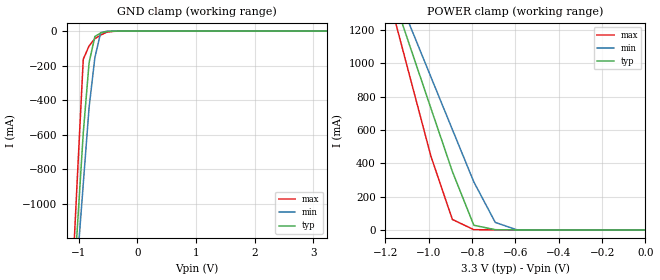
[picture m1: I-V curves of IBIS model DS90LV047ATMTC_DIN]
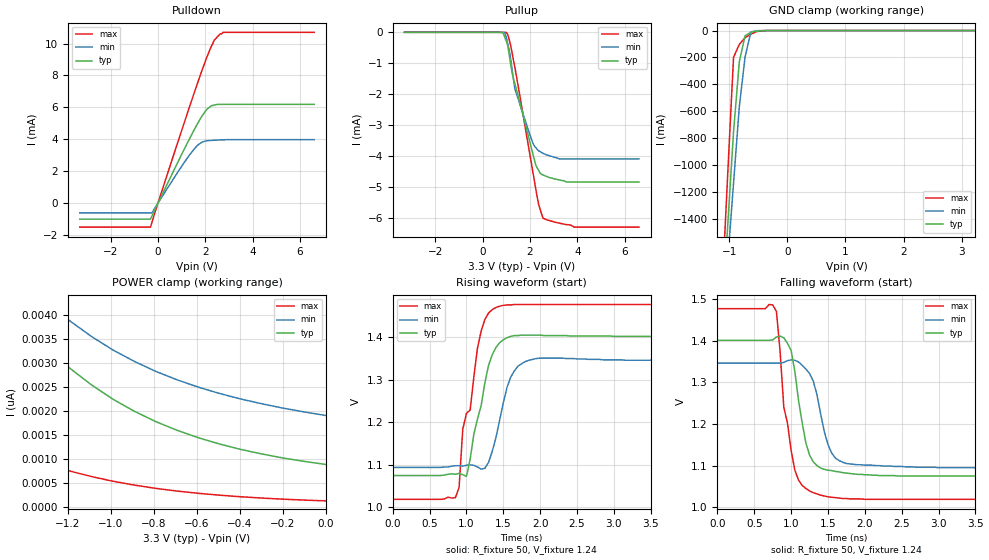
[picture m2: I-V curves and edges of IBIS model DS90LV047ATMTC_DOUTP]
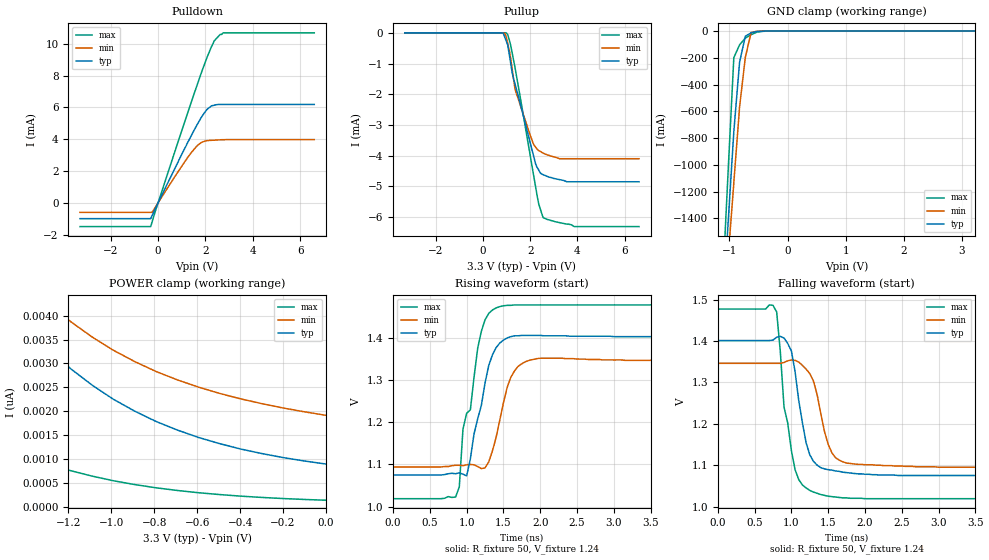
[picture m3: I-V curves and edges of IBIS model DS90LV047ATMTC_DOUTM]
|   National Semiconductor Corporation
|   Interface Products Group
|   IBIS Model of DSLVDS1047
|   16L TSSOP Package
[IBIS Ver]   3.2
[File name]   dslvds1047.ibs
[File Rev]   1.2
[Date]   7/06/04
[Source]   File originated at National Semiconductor Corporation.
   Interface Group/Analog Division. All data based on
   Empirical Measurements(Bench).
[Notes]   File created by DAK.
   Rev 1.1: In Rising Falling Tables, changes Vref
   from 3.3v to 1.2v---milt
   Rev 1.2: a new model based on a spice model simulation
   data - dglisic
[Disclaimer]
(C) Copyright National Semiconductor Corporation 1994
   All rights reserved
   National Semiconductor Corporation hereby grants
the user of this IBIS model a non-exclusive, nontransferable
license to use this IBIS model under the following terms.
Before using this IBIS model, the user should read this
license.  If the user does not accept these terms,  the
IBIS model should be returned to National within 30 days.
   The user is granted this license only to use the
IBIS model and is not granted rights to sell, load, rent,
lease or license the IBIS model in whole or in part, or in
modified form to anyone other than user. User may modify
the IBIS model to suit its specific applications but rights
to derivative works and such modifications shall belong to
National.
   This IBIS model is provided on an "AS IS" basis and
National makes absolutely no warranty with respect to the
information contained herein.NATIONAL DISCLAIMS AND CUSTOMER
WAIVES ALL WARRANTIES, EXPRESS OR IMPLIED, INCLUDING
WARRANTIES OF MERCHANTABILITY OR FITNESS FOR A PARTICULAR
PURPOSE. The entire risk as to quality and performance is
with the Customer. ACCORDINGLY, IN NO EVENT SHALL THE
COMPANY BE LIABLE FOR ANY DAMAGES, WHETHER IN CONTRACT OR
TORT,INCLUDING ANY LOST PROFITS OR OTHER INCIDENTAL,
CONSEQUENTIAL, EXEMPLARY, OR PUNITIVE DAMAGES ARISING OUT
OF THE USE OR APPLICATION OF THE IBIS model provided in
this package.Further, National reserves the right to make
changes without notice to any product herein to improve
reliability, function, or design. National does not convey
any license under patent rights or any other intellectual
property rights, including those of third parties.
   National is not obligated to provide maintenance or support
for the licensed IBIS model.
Contact National at ATTN:INTERFACE APPLICATIONS/IBIS MODELS
   5 Foden Road, M/S 03-03
   South Porltand, ME 04106
   (207) 541-6031
[Copyright]   Copyright 1994, National Semiconductor, All Rights Reserved
[Component]   DSLVDS1047
[Manufacturer]  National Semiconductor Corp
[Package]
|   typ   min   max
R_pkg   91m   78m   115m
L_pkg   2.49n   2.15n   3.12n
C_pkg   0.086p   0.076p   0.109p
[Pin]   signal_name   model_name   R_pin   L_pin   C_pin
1   EN   DS90LV047ATMTC_EN   113m   3.053n   .108p
2   DIN1   DS90LV047ATMTC_DIN   91m   2.494n   .083p
3   DIN2   DS90LV047ATMTC_DIN   80m   2.218n   .079p
4   VDD   POWER   78m   2.157n   .076p
5   GND   GND   79m   2.183n   .077p
6   DIN3   DS90LV047ATMTC_DIN   84m   2.318n   .078p
7   DIN4   DS90LV047ATMTC_DIN   93m   2.550n   .083p
8   EN*   DS90LV047ATMTC_EN   108m   2.984n   .107p
9   DOUT4-   DS90LV047ATMTC_DOUTM  115m   3.121n   .109p
10   DOUT4+   DS90LV047ATMTC_DOUTP   93m   2.551n   .083p
11   DOUT3+   DS90LV047ATMTC_DOUTP   81m   2.237n   .079p
12   DOUT3-   DS90LV047ATMTC_DOUTM   78m   2.152n   .076p
13   DOUT2-   DS90LV047ATMTC_DOUTM   79m   2.173n   .076p
14   DOUT2+   DS90LV047ATMTC_DOUTP   83m   2.291n   .078p
15   DOUT1+   DS90LV047ATMTC_DOUTP   90m   2.480n   .083p
16   DOUT1-   DS90LV047ATMTC_DOUTM  106m   2.914n   .106p
[Diff_pin]   inv_pin   vdiff   tdelay_typ   tdelay_min   tdelay_max
10   9   0.7   0   0   1.7ns
11   12   NA   0   0   0
14   13   NA   0   0   0
15   16   NA   0   0   0
| Models and submodels in the file (4): DS90LV047ATMTC_DIN (Input), DS90LV047ATMTC_EN (Input), DS90LV047ATMTC_DOUTP (3-state), DS90LV047ATMTC_DOUTM (3-state)
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[Model]   DS90LV047ATMTC_DIN
Model_type Input
Vinh=2.0
Vinl=0.8
|   TYP   MIN   MAX
C_comp   3p   3p   3p
[Temperature Range] 25   85   -40
[Voltage Range]   3.30   3.00   3.60
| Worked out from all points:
|   GND clamp passes 1 mA (typ) near -0.44 V on its own axis
|   POWER clamp passes 1 mA (typ) near -0.65 V on its own axis
[GND Clamp]
|V(groundclamp)   I(typ)   I(min)   I(max)
-3.3V     -13.98A    -11.83A    -17.63A
-1.122V   -1.669A    -1.777A    -1.526A
-1.023V   -1.129A    -1.331A    -837mA
-924mV    -590.8mA   -886.6mA   -163.5mA
-825mV    -184mA     -443.7mA   -85.99mA
-726mV    -31.28mA   -153.9mA   -44.23mA
-627mV    -11.3mA    -9.068mA   -22.94mA
-528mV    -2.886mA   -1.123mA   -6.914mA
-330mV    -102.6uA   -43.64uA   -229.3uA
3.234V    1.855uA    1.074uA    3.371uA
[POWER Clamp]
|V(table)   I(typ)   I(min)   I(max)
-3.267V   9.584A     8.291A     11.75A
-1.188V   1.491A     1.55A      1.416A
-1.089V   1.11A      1.233A     928.2mA
-990mV    729.5mA    917.3mA    441.9mA
-891mV    350.5mA    602.3mA    63.05mA
-792mV    28.24mA    288.1mA    1.817mA
-693mV    1.617mA    45.27mA    453.5uA
-594mV    118.9uA    1.221mA    66.77uA
0V        857.1pA    1.83nA     132.3pA
[Model]   DS90LV047ATMTC_DOUTP
Model_type 3-state
Enable Active-High
Polarity Non-Inverting
Vref=1.21
Vmeas=1.21
Rref=50   | 100 Ohms Across Outputs OUTP and OUTM
Cref=0p
|   TYP   MIN   MAX
C_comp   2.5p   2p   3.5p
[Temperature Range] 25   85   -40
[Voltage Range]   3.30   3.00   3.60
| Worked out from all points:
|   slope of the pulldown table from 0 to 0.495 V, typ, clamps not added: 327 ohm
|   GND clamp passes 1 mA (typ) near -0.42 V on its own axis
|   falling waveform, R_fixture 50, V_fixture 1.24: 20-80 % time 184ps typ, 203ps min, 183ps max; typ from 1.4 V to 1.07 V
|   rising waveform, R_fixture 50, V_fixture 1.24: 20-80 % time 231ps typ, 209ps min, 240ps max; typ from 1.07 V to 1.4 V
[Pullup]
|Vtable   I(typ)   I(min)   I(max)
-3.3V     1.3nA      2.13nA     2.37nA
800mV     -1.95uA    -4.2uA     2.12nA
988mV     -265uA     -130uA     1.03nA
1.05V     -391uA     -339uA     -55.9uA
1.175V    -986uA     -810uA     -399uA
1.362V    -1.67mA    -1.84mA    -1.14mA
2.112V    -3.91mA    -3.57mA    -4.49mA
2.238V    -4.29mA    -3.73mA    -5.05mA
2.362V    -4.47mA    -3.84mA    -5.57mA
2.55V     -4.62mA    -3.92mA    -6.02mA
3.862V    -4.85mA    -4.1mA     -6.31mA
6.6V      -4.85mA    -4.1mA     -6.31mA
[Pulldown]
|V(pulldown)   I(typ)   I(min)   I(max)
-3.3V     -1mA       -603uA     -1.5mA
-313mV    -1mA       -603uA     -1.5mA
-250mV    -796uA     -603uA     -1.19mA
875mV     2.67mA     2.03mA     3.98mA
1.625V    4.85mA     3.55mA     7.31mA
1.812V    5.34mA     3.78mA     8.12mA
2V        5.75mA     3.89mA     8.88mA
2.25V     6.1mA      3.93mA     9.81mA
2.375V    6.14mA     3.94mA     10.2mA
2.625V    6.19mA     3.96mA     10.6mA
2.75V     6.19mA     3.97mA     10.7mA
6.6V      6.19mA     3.98mA     10.7mA
[GND Clamp]
|V(groundclamp)   I(typ)   I(min)   I(max)
-3.3V     -17.79A    -15.11A    -22.31A
-1.122V   -2.13A     -2.273A    -1.936A
-1.023V   -1.44A     -1.703A    -1.057A
-924mV    -751.6mA   -1.134A    -198.9mA
-825mV    -232.9mA   -567.3mA   -103.3mA
-726mV    -38.72mA   -196.7mA   -52.72mA
-627mV    -13.96mA   -11.49mA   -27.64mA
-528mV    -3.584mA   -1.412mA   -8.348mA
-330mV    -123.4uA   -52.37uA   -268.9uA
3.234V    857.1pA    2.099nA    93.12pA
[POWER Clamp]
|V(table)   I(typ)   I(min)   I(max)
-3.267V   46.62nA    40.29nA    20.01nA
-2.277V   12.92nA    12.82nA    4.536nA
-2.178V   11.26nA    11.38nA    3.87nA
-1.98V    8.554nA    9.002nA    2.81nA
-1.881V   7.457nA    8.027nA    2.393nA
-1.683V   5.654nA    6.409nA    1.724nA
-1.485V   4.298nA    5.176nA    1.239nA
-1.287V   3.289nA    4.247nA    889pA
-1.089V   2.545nA    3.553nA    639.8pA
-891mV    2.001nA    3.039nA    463.6pA
-495mV    1.32nA     2.372nA    253.7pA
0V        893pA      1.913nA    134.7pA
[Ramp]
|   TYP   MIN   MAX
dV/dt_r   196mV/.233ns   153mV/.244ns   276mV/.211ns
dV/dt_f   196mv/.190ns   153mV/.216ns   276mV/.180ns
R_load=50
[Falling Waveform]
R_fixture=50
V_fixture=1.24
V_fixture_min=1.22
V_fixture_max=1.25
|Time   V(typ)   V(min)   V(max)
0s        1.401V     1.346V     1.477V
800ps     1.409V     1.346V     1.47V
850ps     1.411V     1.346V     1.373V
900ps     1.407V     1.348V     1.24V
1ns       1.376V     1.354V     1.135V
1.1ns     1.256V     1.349V     1.065V
1.25ns    1.125V     1.321V     1.039V
1.5ns     1.089V     1.15V      1.025V
1.7ns     1.083V     1.108V     1.021V
4.95ns    1.075V     1.094V     1.019V
[Rising Waveform]
R_fixture=50
V_fixture=1.24
V_fixture_min=1.22
V_fixture_max=1.25
|Time   V(typ)   V(min)   V(max)
0s        1.075V     1.094V     1.019V
850ps     1.078V     1.098V     1.023V
900ps     1.08V      1.098V     1.047V
1ns       1.073V     1.099V     1.221V
1.05ns    1.113V     1.1V       1.229V
1.15ns    1.208V     1.095V     1.375V
1.4ns     1.376V     1.164V     1.47V
1.6ns     1.402V     1.306V     1.476V
1.85ns    1.405V     1.346V     1.477V
4.95ns    1.401V     1.346V     1.477V
[Model]   DS90LV047ATMTC_DOUTM
Model_type 3-state
Enable Active-High
Polarity Inverting
Vref=1.21
Vmeas=1.21
Rref=50   | 100 Ohms Across Outputs OUTP and OUTM
Cref=0p
|   TYP   MIN   MAX
C_comp   2.5p   2p   3.5p
[Temperature Range] 25   85   -40
[Voltage Range]   3.30   3.00   3.60
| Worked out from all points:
|   slope of the pulldown table from 0 to 0.495 V, typ, clamps not added: 327 ohm
|   GND clamp passes 1 mA (typ) near -0.42 V on its own axis
|   falling waveform, R_fixture 50, V_fixture 1.24: 20-80 % time 184ps typ, 203ps min, 183ps max; typ from 1.4 V to 1.07 V
|   rising waveform, R_fixture 50, V_fixture 1.24: 20-80 % time 231ps typ, 209ps min, 240ps max; typ from 1.07 V to 1.4 V
[Pullup]
|Vtable   I(typ)   I(min)   I(max)
-3.3V     1.3nA      2.13nA     2.37nA
800mV     -1.95uA    -4.2uA     2.12nA
988mV     -265uA     -130uA     1.03nA
1.05V     -391uA     -339uA     -55.9uA
1.175V    -986uA     -810uA     -399uA
1.362V    -1.67mA    -1.84mA    -1.14mA
2.112V    -3.91mA    -3.57mA    -4.49mA
2.238V    -4.29mA    -3.73mA    -5.05mA
2.362V    -4.47mA    -3.84mA    -5.57mA
2.55V     -4.62mA    -3.92mA    -6.02mA
3.862V    -4.85mA    -4.1mA     -6.31mA
6.6V      -4.85mA    -4.1mA     -6.31mA
[Pulldown]
|V(pulldown)   I(typ)   I(min)   I(max)
-3.3V     -1mA       -603uA     -1.5mA
-313mV    -1mA       -603uA     -1.5mA
-250mV    -796uA     -603uA     -1.19mA
875mV     2.67mA     2.03mA     3.98mA
1.625V    4.85mA     3.55mA     7.31mA
1.812V    5.34mA     3.78mA     8.12mA
2V        5.75mA     3.89mA     8.88mA
2.25V     6.1mA      3.93mA     9.81mA
2.375V    6.14mA     3.94mA     10.2mA
2.625V    6.19mA     3.96mA     10.6mA
2.75V     6.19mA     3.97mA     10.7mA
6.6V      6.19mA     3.98mA     10.7mA
[GND Clamp]
|V(groundclamp)   I(typ)   I(min)   I(max)
-3.3V     -17.79A    -15.11A    -22.31A
-1.122V   -2.13A     -2.273A    -1.936A
-1.023V   -1.44A     -1.703A    -1.057A
-924mV    -751.6mA   -1.134A    -198.9mA
-825mV    -232.9mA   -567.3mA   -103.3mA
-726mV    -38.72mA   -196.7mA   -52.72mA
-627mV    -13.96mA   -11.49mA   -27.64mA
-528mV    -3.584mA   -1.412mA   -8.348mA
-330mV    -123.4uA   -52.37uA   -268.9uA
3.234V    857.1pA    2.099nA    93.12pA
[POWER Clamp]
|V(table)   I(typ)   I(min)   I(max)
-3.267V   46.62nA    40.29nA    20.01nA
-2.277V   12.92nA    12.82nA    4.536nA
-2.178V   11.26nA    11.38nA    3.87nA
-1.98V    8.554nA    9.002nA    2.81nA
-1.881V   7.457nA    8.027nA    2.393nA
-1.683V   5.654nA    6.409nA    1.724nA
-1.485V   4.298nA    5.176nA    1.239nA
-1.287V   3.289nA    4.247nA    889pA
-1.089V   2.545nA    3.553nA    639.8pA
-891mV    2.001nA    3.039nA    463.6pA
-495mV    1.32nA     2.372nA    253.7pA
0V        893pA      1.913nA    134.7pA
[Ramp]
|   TYP   MIN   MAX
dV/dt_r   196mV/.233ns   153mV/.244ns   276mV/.211ns
dV/dt_f   196mv/.190ns   153mV/.216ns   276mV/.180ns
R_load=50
[Falling Waveform]
R_fixture=50
V_fixture=1.24
V_fixture_min=1.22
V_fixture_max=1.25
|Time   V(typ)   V(min)   V(max)
0s        1.401V     1.346V     1.477V
800ps     1.409V     1.346V     1.47V
850ps     1.411V     1.346V     1.373V
900ps     1.407V     1.348V     1.24V
1ns       1.376V     1.354V     1.135V
1.1ns     1.256V     1.349V     1.065V
1.25ns    1.125V     1.321V     1.039V
1.5ns     1.089V     1.15V      1.025V
1.7ns     1.083V     1.108V     1.021V
4.95ns    1.075V     1.094V     1.019V
[Rising Waveform]
R_fixture=50
V_fixture=1.24
V_fixture_min=1.22
V_fixture_max=1.25
|Time   V(typ)   V(min)   V(max)
0s        1.075V     1.094V     1.019V
850ps     1.078V     1.098V     1.023V
900ps     1.08V      1.098V     1.047V
1ns       1.073V     1.099V     1.221V
1.05ns    1.113V     1.1V       1.229V
1.15ns    1.208V     1.095V     1.375V
1.4ns     1.376V     1.164V     1.47V
1.6ns     1.402V     1.306V     1.476V
1.85ns    1.405V     1.346V     1.477V
4.95ns    1.401V     1.346V     1.477V
